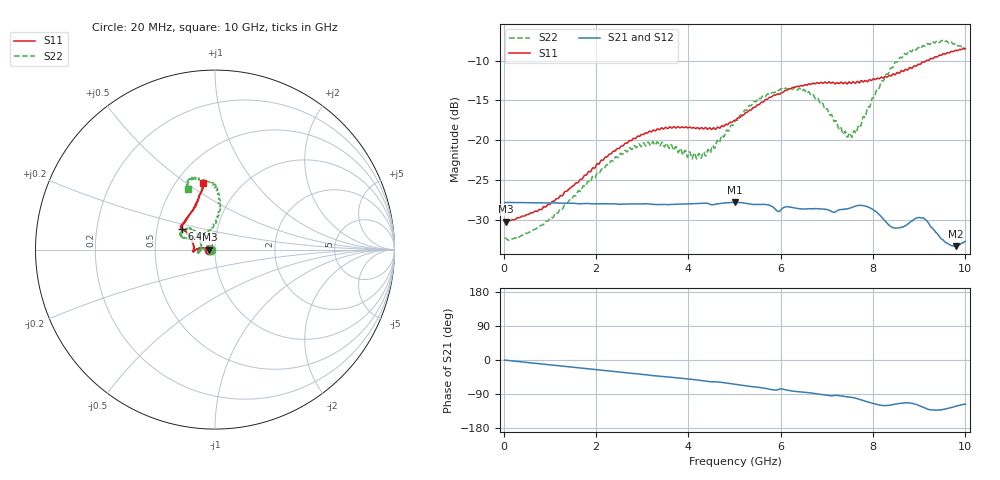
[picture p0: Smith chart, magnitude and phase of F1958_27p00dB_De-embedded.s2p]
! Integrated Device Technology
! Corporate Headquarters
! 6024 Silver Creek Valley Road
! San Jose, CA 95138  USA
! Phone:  1-408-284-8200
! Toll Free:  1-800-223-1366
! Webpage:  http://www.idt.com/
! Timing and RF Division
! 515 Groton Road, Suite 102
! Westford, MA 01886-6024
! Device:  F1958
! Description: 7-bit 0.25 dB Digital Step Attenuator
! Frequency:  0.001 -  6.000 GHz
! Package:  4x4 mm Thin QFN Plastic Package: 24 pin
! Ports:  2 RF, 12 DC
!  Pin  1  = D0
!  Pin  2  = VDD
!  Pin  3  = VMODE
!  Pin  4  = GND
!  Pin  5  = RF1  =  Port 1
!  Pin  6  = GND
!  Pin  7  = GND
!  Pin  8  = GND
!  Pin  9  = GND
!  Pin 10  = GND
!  Pin 11  = GND
!  Pin 12  = GND
!  Pin 13  = GND
!  Pin 14  = RF2  =  Port 2
!  Pin 15  = GND
!  Pin 16  = LE
!  Pin 17  = CLK
!  Pin 18  = DATA
!  Pin 19  = D6
!  Pin 20  = D5
!  Pin 21  = D4
!  Pin 22  = D3
!  Pin 23  = D2
!  Pin 24  = D1
! State:  108
! Atten State:  27.00 dB
! Voltage:  +3.30 Volts
! Current:  0.258 mA
! Data:  The device was measured on a F1958 evaluation board which has
!  individual transmission lines to the RF pins.  Data was collected
!  using a calibrated network analyzer.  The evaluation board was
!  de-embedded using Automatic Fixture Removal (AFR).
!  The reference plane is the edge of the package pin.
! Misc:
!  Action Tracker AT0419
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# GHz S dB R 50
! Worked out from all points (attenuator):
!   500 points, 20 MHz to 10 GHz, reference 50 ohm
!   highest |S21| = -27.76 dB at 5 GHz (marker M1); lowest = -33.3 dB at 9.8 GHz (marker M2)
!   lowest |S11| = -30.2 dB at 40 MHz (marker M3), VSWR 1.06, Z = 47 - j0.0426 ohm
!   |S11| at or under -10 dB: start of sweep to 9.156 GHz; 9.199135 GHz to 9.20014 GHz (1.005 MHz wide, 0.0109 % of centre)
!   |S22| runs from -32.5 to -7.5 dB; largest |S21 - S12| = 0.00027
!   S11 on the Smith chart (normalised r, x): 20 MHz: 0.94, -0.00; 6.4 GHz: 0.67, +0.16; 10 GHz: 0.68, +0.58
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0.02  -30.14 -178.9  -27.80 -0.2  -27.79 -0.2  -32.27 -178.9
0.04  -30.17 -179.2  -27.78 -0.5  -27.78 -0.5  -32.23 -178.3
0.84  -28.52 170.8  -27.83 -10.7  -27.82 -10.7  -30.61 172.3
1.7  -24.84 170.8  -27.93 -21.3  -27.92 -21.3  -25.95 171.4
2.62  -20.42 176.9  -27.98 -32.8  -27.96 -32.8  -21.26 -179.4
3.36  -18.65 -175.8  -28.03 -42.4  -28.04 -42.6  -20.54 -169.2
4.24  -18.58 -179.1  -27.89 -53.4  -27.89 -53.5  -21.68 169.1
4.5  -18.64 175.0  -28.07 -57.4  -28.07 -57.4  -21.04 151.4
5  -17.50 161.4  -27.76 -63.9  -27.78 -64.0  -17.67 137.1
5.02  -17.50 160.6  -27.77 -64.2  -27.78 -64.3  -17.43 138.1
5.58  -15.23 150.4  -28.03 -73.0  -28.04 -73.1  -14.68 139.9
6.4  -13.25 147.8  -28.56 -84.0  -28.58 -83.9  -13.45 155.9
6.68  -12.89 146.6  -28.56 -87.3  -28.58 -87.1  -14.38 158.0
7.5  -12.74 138.3  -28.48 -97.9  -28.48 -97.8  -19.07 120.2
7.68  -12.70 135.3  -28.16 -102.8  -28.15 -102.7  -18.12 99.7
7.9  -12.51 128.9  -28.36 -111.3  -28.34 -111.2  -15.80 89.3
8.34  -11.88 118.8  -30.58 -119.7  -30.58 -119.8  -11.54 83.9
8.66  -11.39 113.1  -30.84 -113.5  -30.81 -113.5  -9.30 87.7
9.08  -10.16 107.1  -29.70 -124.5  -29.71 -124.5  -8.12 98.9
9.52  -9.14 101.7  -32.49 -130.3  -32.55 -130.4  -7.64 109.3
9.8  -8.73 100.7  -33.25 -121.6  -33.26 -121.5  -7.89 112.9
10  -8.52 99.9  -32.65 -116.9  -32.66 -116.7  -8.64 114.0
